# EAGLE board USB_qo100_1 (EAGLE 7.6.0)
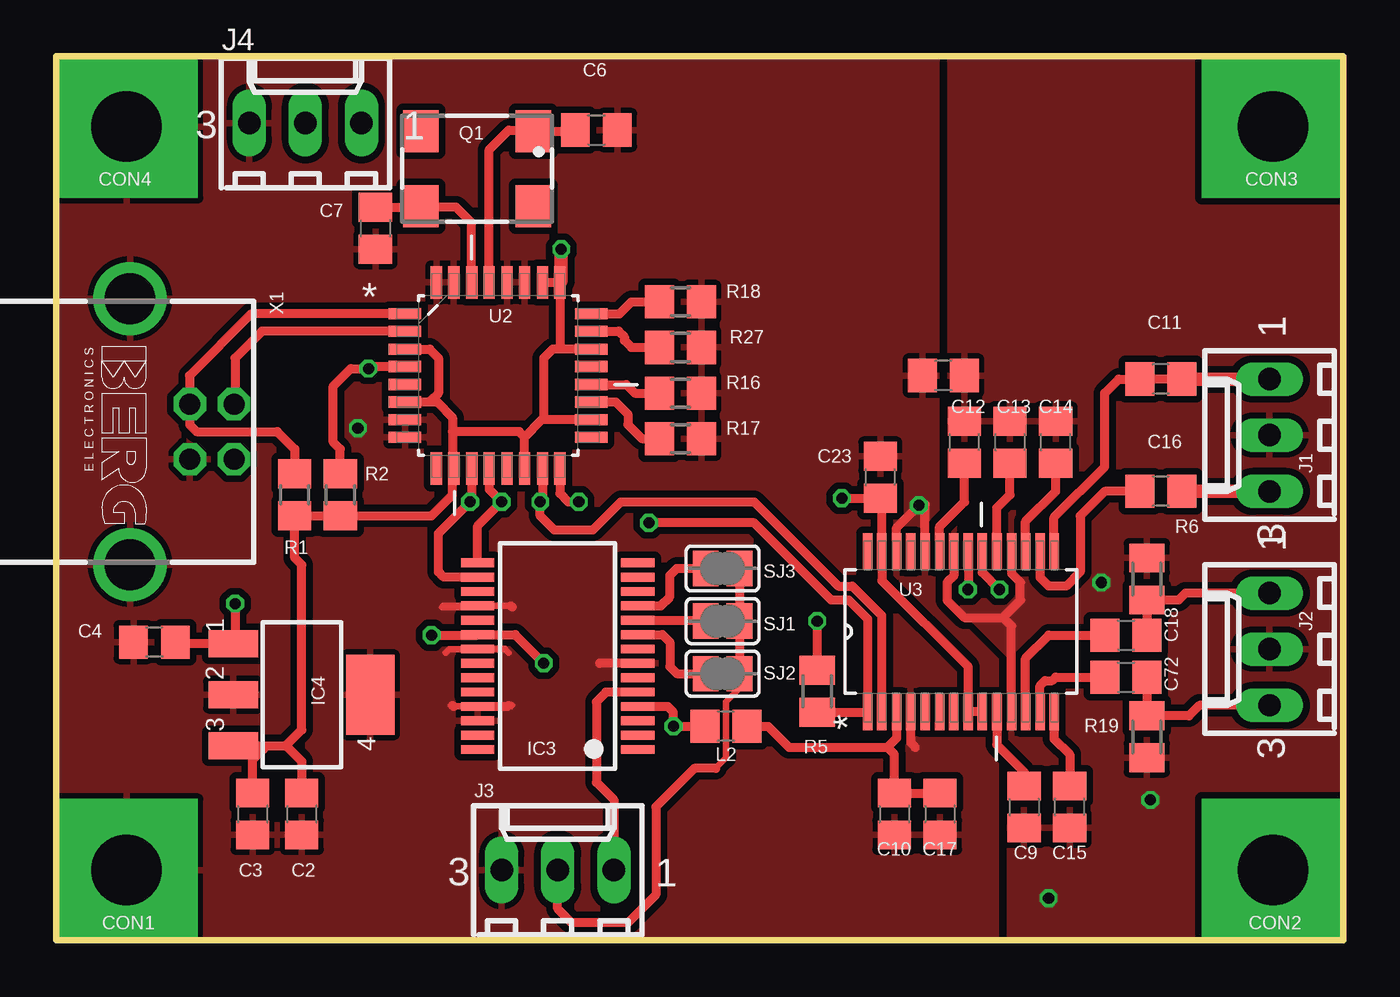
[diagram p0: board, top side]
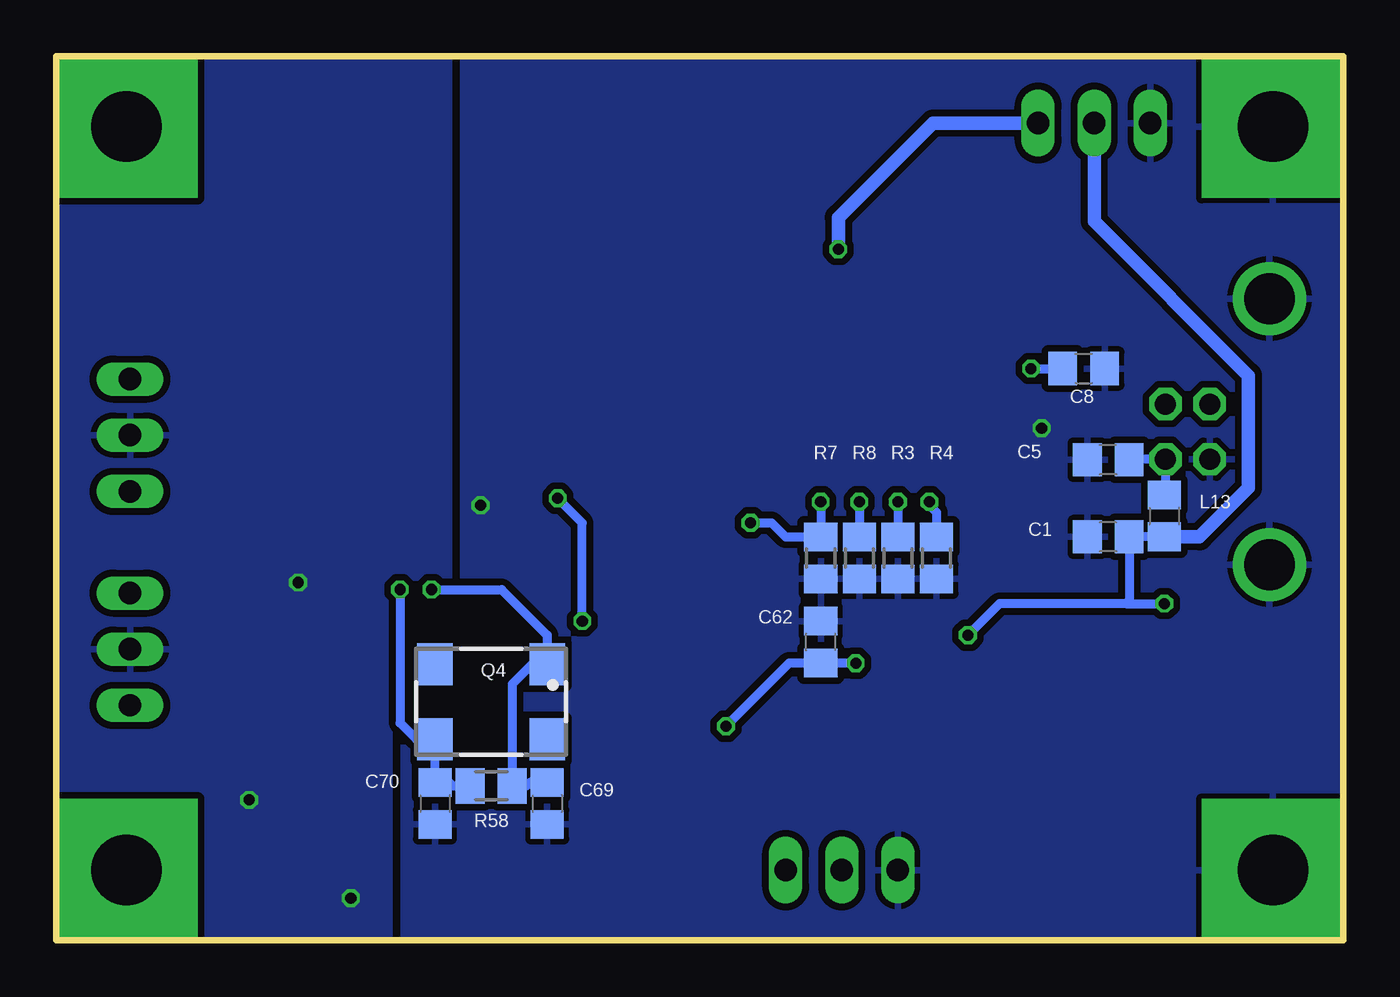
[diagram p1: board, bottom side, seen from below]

Size 58.26 x 40.01 mm. Coordinates in mm from the lower left corner, seen from the top.
Outline: 0,0 0,40.01 58.26,40.01 58.26,0 0,0
Copper layers (1*16): Top 0.035mm / dielectric 1.5mm / Bottom 0.035mm
Design rules "SeeedStudio_2layer_DRU_no_angle_20140221 *": minimum track width 6mil, minimum drill 12mil, track to track 6mil, track to pad 6mil, pad to pad 6mil, via to via 6mil, smd to smd 0mil, copper to edge 0mil, drill to drill 10mil, minimum pad ring 10mil, minimum via ring 6mil, stop-mask expansion 2mil, vias tented up to drill 100mil, thermal gap 10mil

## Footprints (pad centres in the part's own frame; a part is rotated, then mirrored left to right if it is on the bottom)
C0805 = smd 1.3 x 1.5: 1 -0.95,0; 2 0.95,0
HOLE3 = drill 3.2 pad 6.452 square: 1 0,0
SSOP28 = smd 0.4 x 1.5: 1 -4.225,-3.625; 2 -3.575,-3.625; 3 -2.925,-3.625; 4 -2.275,-3.625; 5 -1.625,-3.625; 6 -0.975,-3.625; 7 -0.325,-3.625; 8 0.325,-3.625; 9 0.975,-3.625; 10 1.625,-3.625; 11 2.275,-3.625; 12 2.925,-3.625; 13 3.575,-3.625; 14 4.225,-3.625; 15 4.225,3.625; 16 3.575,3.625; 17 2.925,3.625; 18 2.275,3.625; 19 1.625,3.625; 20 0.975,3.625; 21 0.325,3.625; 22 -0.325,3.625; 23 -0.975,3.625; 24 -1.625,3.625; 25 -2.275,3.625; 26 -2.925,3.625; 27 -3.575,3.625; 28 -4.225,3.625
SOT223 = smd 1.219 x 2.235: 1 -2.311,-3.099; 2 0,-3.099; 3 2.311,-3.099 | smd 3.6 x 2.2: 4 0,3.099
6410-03 = drill 1.016 long: 1 2.54,0; 2 0,0; 3 -2.54,0
CRYSTAL_5X7 = smd 1.6 x 1.9: 1 -2.55,-1.7; 2 2.55,-1.7; 3 2.55,1.7; 4 -2.55,1.7
R0805 = smd 1.3 x 1.5: 1 -0.95,0; 2 0.95,0
M0805 = smd 1.3 x 1.6: 1 -0.95,0; 2 0.95,0
SJ = smd 1.168 x 1.6: 1 -0.762,0; 2 0.762,0
QFP80P900X900X145-32N = smd 1.473 x 0.508: 1 -4.216,2.794; 2 -4.216,2.007; 3 -4.216,1.194; 4 -4.216,0.406; 5 -4.216,-0.406; 6 -4.216,-1.194; 7 -4.216,-2.007; 8 -4.216,-2.794; 17 4.216,-2.794; 18 4.216,-2.007; 19 4.216,-1.194; 20 4.216,-0.406; 21 4.216,0.406; 22 4.216,1.194; 23 4.216,2.007; 24 4.216,2.794 | smd 0.508 x 1.473: 9 -2.794,-4.216; 10 -2.007,-4.216; 11 -1.194,-4.216; 12 -0.406,-4.216; 13 0.406,-4.216; 14 1.194,-4.216; 15 2.007,-4.216; 16 2.794,-4.216; 25 2.794,4.216; 26 2.007,4.216; 27 1.194,4.216; 28 0.406,4.216; 29 -0.406,4.216; 30 -1.194,4.216; 31 -2.007,4.216; 32 -2.794,4.216
SOP65P780X200-28N = smd 1.651 x 0.432: 1 -3.632,4.216; 2 -3.632,3.581; 3 -3.632,2.921; 4 -3.632,2.286; 5 -3.632,1.626; 6 -3.632,0.965; 7 -3.632,0.33; 8 -3.632,-0.33; 9 -3.632,-0.965; 10 -3.632,-1.626; 11 -3.632,-2.286; 12 -3.632,-2.921; 13 -3.632,-3.581; 14 -3.632,-4.216; 15 3.632,-4.216; 16 3.632,-3.581; 17 3.632,-2.921; 18 3.632,-2.286; 19 3.632,-1.626; 20 3.632,-0.965; 21 3.632,-0.33; 22 3.632,0.33; 23 3.632,0.965; 24 3.632,1.626; 25 3.632,2.286; 26 3.632,2.921; 27 3.632,3.581; 28 3.632,4.216
PN61729-S = drill 0.95 octagon: 1 1.25,4.71; 2 -1.25,4.71; 3 -1.25,2.71; 4 1.25,2.71 | drill 2.3 pad 2.9: S1 -6.02,0; S2 6.02,0

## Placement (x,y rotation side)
C1  100n  [C0805]  10.64,18.26 180 bottom
C2  100n  [C0805]  11.11,5.71 270 top
C3  10u  [C0805]  8.89,5.71 270 top
C4  10u  [C0805]  4.45,13.49 180 top
C5  100n  [C0805]  10.64,21.75 180 bottom
C6  22p  [C0805]  24.45,36.67 0 top
C7  22p  [C0805]  14.45,32.23 270 top
C8  100n  [C0805]  11.75,25.88 0 bottom
C9  10u  [C0805]  43.81,6.03 270 top
C10  10u  [C0805]  37.94,5.71 270 top
C11  100n  [C0805]  50.01,25.4 180 top
C12  1u  [C0805]  41.12,22.54 90 top
C13  1u  [C0805]  43.18,22.54 90 top
C14  1u  [C0805]  45.24,22.54 90 top
C15  10u  [C0805]  45.88,6.03 90 top
C16  100n  [C0805]  50.01,20.32 180 top
C17  100n  [C0805]  40.01,5.71 270 top
C18  100n  [C0805]  48.42,13.81 0 top
C23  1u  [C0805]  37.31,20.95 90 top
C62  100n  [C0805]  23.65,13.49 90 bottom
C69  22p  [C0805]  36.04,6.19 270 bottom
C70  22p  [C0805]  41.12,6.19 270 bottom
C72  100n  [C0805]  48.42,11.91 0 top
CON1  [HOLE3]  3.17,3.17 0 top
CON2  [HOLE3]  55.09,3.17 0 top
CON3  [HOLE3]  55.09,36.83 0 top
CON4  [HOLE3]  3.17,36.83 0 top
IC3  FT232RL  [SSOP28]  22.7,12.86 90 top
IC4  UA78M33CDCY  [SOT223]  11.11,11.11 270 top
J1  Audio Output  [6410-03]  54.93,22.86 90 top
J2  Audio Input  [6410-03]  54.93,13.18 90 top
J3  PTT_RX  [6410-03]  22.7,3.17 0 top
J4  SV  [6410-03]  11.27,36.99 0 top
L2  100uH  [C0805]  30.32,9.68 180 top
L3  100uH  [C0805]  40.16,25.56 180 top
L13  100uH  [C0805]  8.1,19.21 270 bottom
Q1  6MHz  [CRYSTAL_5X7]  19.05,34.92 180 top
Q4  12MHz  [CRYSTAL_5X7]  38.58,10.79 180 bottom
R1  1k5  [R0805]  10.79,20.16 270 top
R2  10k  [R0805]  12.86,20.16 270 top
R3  15k  [R0805]  20.16,17.3 90 bottom
R4  15k  [R0805]  18.41,17.3 90 bottom
R5  1k5  [M0805]  34.45,11.27 90 top
R6  22k  [M0805]  49.37,16.35 270 top
R7  15k  [R0805]  23.65,17.3 90 bottom
R8  15k  [R0805]  21.91,17.3 90 bottom
R16  15k  [R0805]  28.26,24.77 180 top
R17  15k  [R0805]  28.26,22.7 180 top
R18  15k  [R0805]  28.26,28.89 180 top
R19  22k  [M0805]  49.37,9.21 90 top
R27  15k  [R0805]  28.26,26.83 180 top
R58  1M  [M0805]  38.58,6.99 180 bottom
SJ1  [SJ]  30.16,14.45 0 top
SJ2  [SJ]  30.16,12.06 0 top
SJ3  [SJ]  30.16,16.83 0 top
U2  TUSB2046BVF  [QFP80P900X900X145-32N]  20,25.56 0 top
U3  PCM2906BDB  [SOP65P780X200-28N]  40.96,13.97 90 top
X1  PN61729-S  [PN61729-S]  3.33,23.02 270 top

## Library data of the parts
C1-C18 C23 C62 C69 C70 C72 R1-R8 R16-R19 R27 R58 = rcl
CON1-CON4 = lindenau
IC3 = ftdichip; MPN: FT232RL; OC_FARNELL: 1146032; OC_NEWARK: 91K9918
IC4 = linear
J1-J4 = con-molex; OC_FARNELL: unknown; OC_NEWARK: unknown
L2 L3 L13 Q1 Q4 = Jochen
SJ1-SJ3 = jumper
U2 = Texas Instruments_By_element14_Batch_1; MPN: TUSB2046BVF; OC_FARNELL: 1470507; OC_NEWARK: 77C1805; PACKAGE: LQFP-32; SUPPLIER: TEXAS INSTRUMENTS
U3 = Texas Instruments_By_element14_Batch_1; MPN: PCM2906BDB; OC_FARNELL: -; OC_NEWARK: 51P6653; PACKAGE: SSOP-28; SUPPLIER: Texas Instruments
X1 = con-berg; OC_FARNELL: unknown; OC_NEWARK: unknown

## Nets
+3V3: C2.1 C3.1 IC4.3 J4.1 R1.2 R2.2 U2.3 U2.6 U2.10 U2.14 U2.18 U2.22 U2.25 U2.26
+5V: C1.1 C4.1 C62.1 IC3.4 IC3.20 IC4.1 J4.2 L2.2 L13.2
AGND: C9.2 C12.2 C13.2 C14.2 C15.1 J1.2 J2.2 L3.1 R6.1 R19.1 U3.11 U3.18 U3.22
GND: C1.2 C2.2 C3.2 C4.2 C5.2 C6.2 C7.2 C8.2 C10.2 C17.2 C23.2 C62.2 C69.2 C70.2 CON1.1 CON4.1 IC3.7 IC3.18 IC3.21 IC3.25 IC3.26 IC4.2 IC4.4 J3.3 J4.3 L3.2 R3.1 R4.1 R7.1 R8.1 R16.1 R17.1 R18.1 R27.1 U2.7 U2.8 U2.27 U2.28 U2.31 U2.32 U3.4 U3.24 U3.26 X1.4 X1.S1 X1.S2
N$1: C5.1 L13.1 X1.1
N$2: U2.2 X1.2
N$3: IC3.10 SJ1.1
N$4: C7.1 Q1.3 U2.30
N$5: C11.2 U3.15
N$6: C6.1 Q1.1 U2.29
N$7: C72.2 J2.3 R19.2
N$8: IC3.9 SJ2.1
N$9: C8.1 R2.1 U2.4
N$10: R1.1 U2.1 X1.3
N$11: IC3.11 SJ3.1
N$12: C16.2 U3.16
N$13: C18.1 U3.12
N$14: C18.2 J2.1 R6.2
N$15: C11.1 J1.1
N$16: C16.1 J1.3
N$25: IC3.5 J3.1
N$70: C72.1 U3.13
N$73: C69.1 Q4.1 R58.1 U3.21
N$74: C9.1 U3.10
N$75: C14.1 U3.17
N$76: C13.1 U3.19
N$77: C12.1 U3.23
N$78: C23.1 R5.2 U3.8 U3.9 U3.27
N$79: C70.1 Q4.3 R58.2 U3.20
N$81: C15.2 U3.14
PTT: J3.2 SJ1.2 SJ2.2 SJ3.2
U_PCM: C10.1 C17.1 L2.1 U3.3
USB1+: IC3.15 R3.2 U2.12
USB1-: IC3.16 R4.2 U2.11
USB2+: R5.1 R7.2 U2.16 U3.1
USB2-: R8.2 U2.15 U3.2
USB3+: R16.2 U2.20
USB3-: R17.2 U2.19
USB4+: R18.2 U2.24
USB4-: R27.2 U2.23

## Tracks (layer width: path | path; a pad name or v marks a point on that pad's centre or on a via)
+3V3  (via drill 0.5)
  Top 0.406: IC4.3 9.21,8.8 | 9.21,8.8 10.39,8.8 | 10.39,8.8 11.11,9.53 11.11,16.99 10.79,17.3 R1.2 R2.2 16.99,19.21 17.94,20.16 17.94,21.29 U2.10 17.94,21.4 17.94,23.02 | U2.3 16.9,26.75 17.3,26.35 17.3,24.77 16.9,24.36 | U2.6 16.9,24.36 | 16.9,24.36 17.23,24.36 17.94,23.65 17.94,23.02 | U2.14 21.2,22.78 | 21.2,22.78 20.95,23.02 17.94,23.02 | U2.18 21.97,23.55 | 21.97,23.55 21.2,22.78 | U2.22 22.86,26.75 | 22.86,26.75 22.47,26.75 22.07,26.35 22.07,23.65 21.97,23.55 | 22.86,26.75 22.8,26.82 U2.25 U2.26 | 10.39,8.8 10.41,8.8 11.11,8.1 C2.1 | 9.21,8.8 9.37,8.64 8.89,8.17 C3.1
  Top 0.61: v22.86,31.27 22.86,29.84 U2.25
  Bottom 0.61: J4.1 18.57,36.99 22.86,32.7 v22.86,31.27
+5V  (via drill 0.5)
  Top 0.406: v16.99,13.81 19.05,13.81 IC3.20 20.77,13.83 v22.07,12.54 | L2.2 v27.94,9.68 27.94,10.32 27.68,10.58 IC3.4 | v8.1,15.24 8.1,13.51 IC4.1 5.46,13.42 C4.1
  Bottom 0.406: 9.84,15.24 15.56,15.24 v16.99,13.81 | v22.07,12.54 C62.1 25.08,12.54 v27.94,9.68 | L13.2 C1.1 9.69,15.4 9.84,15.24 | 9.84,15.24 v8.1,15.24
  Bottom 0.61: L13.2 6.51,18.26 4.29,20.48 4.29,25.56 11.27,32.54 J4.2
AGND  (via drill 0.5)
  Top 0.406: U3.22 40.63,16.5 40.32,16.19 40.32,15.4 41.12,14.61 42.86,14.61 | 42.86,14.61 43.66,15.4 43.66,16.19 43.24,16.61 U3.18 | U3.11 43.24,14.22 42.86,14.61
  other vias: 44.93,1.91 49.53,6.35 47.31,16.19
  pour Top (isolate 0.305): 43.18,0 43.18,12.86 40.48,15.56 40.48,40.01 58.26,40.01 58.26,0
  pour Bottom (isolate 0.305): 43.18,0 43.18,12.86 40.48,15.56 40.48,40.01 58.26,40.01 58.26,0
GND  (via drill 0.5)
  Top 0.305: 17.99,10.58 20.59,10.58 20.64,10.64 | IC3.21 20.31,13.18 20.32,13.18 | 20.48,13.02 20.32,13.18 | 20.32,13.18 17.78,13.18 17.62,13.02 | 20.59,15.13 IC3.18 | IC3.18 17.52,15.13 17.46,15.08 19.02,15.08 IC3.18
  Top 0.406: U3.24 39.33,19.72 v39.05,19.68 38.04,18.67 U3.26 | U3.4 38.67,8.95 38.89,8.73 | IC3.7 24.61,12.53 24.61,12.54 | 20.59,15.13 20.64,15.08 | 17.99,10.58 17.94,10.64 | IC3.25 20.43,10.58 20.48,10.64
  other vias: 13.65,23.18
  pour Bottom (isolate 0.305): 0,0 0,40.01 39.85,40.01 39.85,15.4 42.55,12.7 42.55,0
  pour Top (isolate 0.305): 0,0 0,40.01 39.85,40.01 39.85,15.4 42.55,12.7 42.55,0
N$1
  Bottom 0.406: C5.1 9.67,21.77 X1.1 8.04,20.21 L13.1
N$2
  Top 0.406: U2.2 9.31,27.57 8.1,26.35 8.1,24.32 X1.2
N$3
  Top 0.406: IC3.10 29.36,14.48 SJ1.1
N$4
  Top 0.406: U2.30 18.81,32.47 18.1,33.18 16.55,33.18 Q1.3 16.45,33.18 C7.1
N$5
  Top 0.406: U3.15 45.17,19.14 47.47,21.43 47.47,24.77 48.1,25.4 C11.2 50.64,25.4
N$6
  Top 0.406: U2.29 19.6,35.79 20.48,36.67 21.55,36.67 Q1.1 23.45,36.62 C6.1
N$7
  Top 0.406: J2.3 51.75,10.64 51.28,10.16 R19.2 C72.2
N$8
  Top 0.406: IC3.9 27.44,13.83 27.78,13.49 27.78,12.38 28.1,12.06 SJ2.1
N$9  (via drill 0.5)
  Top 0.406: U2.4 14.22,25.96 v14.13,25.88 13.34,25.88 12.54,25.08 12.54,22.54 12.86,22.23 R2.1
  Bottom 0.406: v14.13,25.88 C8.1
N$10
  Top 0.406: U2.1 8.83,28.35 6.03,25.56 X1.3 6.04,23.32 6.35,23.02 10,23.02 10.79,22.23 R1.1
N$11
  Top 0.406: IC3.11 27.36,15.13 27.78,15.56 27.78,16.51 28.1,16.83 SJ3.1
N$12
  Top 0.406: C16.2 47.47,20.32 46.35,19.21 46.35,16.67 45.72,16.03 44.93,16.03 44.54,16.42 U3.16
N$13
  Top 0.406: U3.12 43.88,12.76 44.93,13.81 C18.1
N$14
  Top 0.406: J2.1 51.12,15.72 50.8,15.4 R6.2 C18.2
N$15
  Top 0.61: C11.1 J1.1
N$16
  Top 0.61: C16.1 J1.3
N$25
  Top 0.406: IC3.5 24.89,11.23 24.45,10.79 24.45,7.14 25.24,6.35 J3.1
N$70
  Top 0.406: U3.13 44.54,11.52 44.77,11.75 45.09,11.75 45.24,11.91 C72.1
N$73  (via drill 0.5)
  Top 0.406: U3.21 41.29,15.89 v41.27,15.88
  Bottom 0.406: v41.27,15.88 38.1,15.88 36.04,13.81 36.04,12.51 | 36.04,12.51 Q4.1 | C69.1 36.83,7.14 36.99,6.99 R58.1 37.62,11.59 36.71,12.51 36.04,12.51
N$74
  Top 0.406: U3.10 42.58,8.85 43.81,7.62 C9.1
N$75
  Top 0.406: U3.17 43.88,18.95 45.24,20.32 C14.1
N$76
  Top 0.406: U3.19 42.58,19.56 43.18,20.16 C13.1
N$77
  Top 0.406: U3.23 39.99,18.72 41.12,19.84 C12.1
N$78  (via drill 0.5)
  Top 0.406: U3.9 U3.8 41.29,12.37 37.38,16.28 U3.27 37.38,19.93 C23.1 v35.56,20 | R5.2 v34.45,14.45
  Bottom 0.406: v34.45,14.45 34.45,18.89 v35.56,20
N$79  (via drill 0.5)
  Top 0.406: U3.20 41.92,16.66 v42.7,15.88
  Bottom 0.406: v42.7,15.88 42.7,9.84 41.96,9.1 Q4.3 C70.1 40.48,7.14 40.32,6.99 R58.2
N$81
  Top 0.406: U3.14 45.17,9.12 45.88,8.41 C15.2
PTT
  Top 0.305: SJ2.2 30.92,11.4 30.32,10.79 30.32,8.26 29.84,7.78
  Top 0.406: SJ3.2 SJ1.2 SJ2.2 | 29.84,7.78 28.89,7.78 27.15,6.03 27.15,2.06 25.88,0.79 23.34,0.79 22.7,1.43 J3.2
U_PCM
  Top 0.406: L2.1 32.23,9.68 33.18,8.73 37.62,8.73 | 37.62,8.73 38.04,9.14 U3.3 | 37.62,8.73 37.94,8.41 C10.1 C17.1
USB1+  (via drill 0.5)
  Top 0.406: U2.12 19.6,20.41 v20.16,19.84 19.08,18.76 IC3.15
  Bottom 0.406: v20.16,19.84 R3.2
USB1-  (via drill 0.5)
  Top 0.406: U2.11 18.81,19.92 v18.73,19.84 17.3,18.41 17.3,16.67 17.54,16.43 IC3.16
  Bottom 0.406: v18.73,19.84 18.73,19.68 18.41,19.37 R4.2
USB2+  (via drill 0.5)
  Top 0.406: U2.16 22.8,20.23 23.18,19.84 v23.65,19.84 | v26.83,18.89 31.59,18.89 35.08,15.4 35.88,15.4 36.74,14.54 U3.1 36.73,10.32 R5.1
  Bottom 0.406: v23.65,19.84 R7.2 25.24,18.26 25.88,18.89 v26.83,18.89
USB2-  (via drill 0.5)
  Top 0.406: U2.15 22.01,19.95 v21.91,19.84 21.91,19.21 22.54,18.57 24.29,18.57 25.56,19.84 31.59,19.84 35.4,16.03 36.04,16.03 37.38,14.69 U3.2
  Bottom 0.406: v21.91,19.84 R8.2
USB3+
  Top 0.406: U2.20 25.81,25.15 26.19,24.77 R16.2
USB3-
  Top 0.406: U2.19 25.32,24.36 25.88,23.81 25.88,23.34 26.51,22.7 R17.2
USB4+
  Top 0.406: U2.24 25.5,28.35 26.04,28.89 R18.2
USB4-
  Top 0.406: U2.23 25.46,27.57 25.72,27.3 25.72,27.15 26.04,26.83 R27.2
